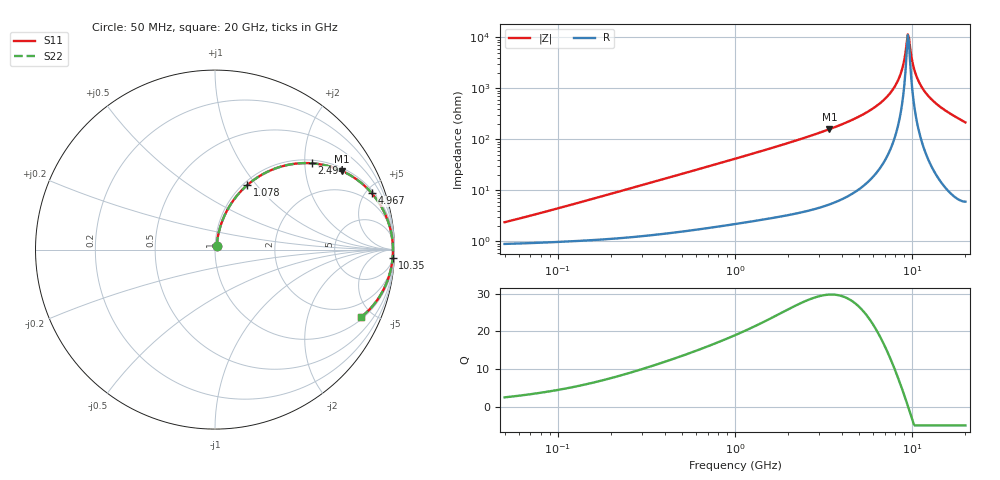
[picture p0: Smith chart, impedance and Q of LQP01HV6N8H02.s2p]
!Murata Part Number: LQP01HV6N8H02
!These Parameters are Measured in Series Mode Connection
!  o--[Z]--o
!Port1  Port2
!  o-------o
!Freq. Start=50[MHz] Stop=20[GHz], 401[Steps]
# Hz S RI R 50
!Freq.(Hz) S11(Real) S11(Imag) S21(Real) S21(Imag) S12(Real) S12(Imag) S22(Real) S22(Imag)
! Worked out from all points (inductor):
!   401 points, 50 MHz to 20 GHz, reference 50 ohm
!   read as one part in series: L = 6.94 nH near 62.6 MHz
!   highest Q = 29.8 at 3.415 GHz (marker M1), where L = 7.36 nH
!   self-resonance near 9.457 GHz
!   S11 on the Smith chart (normalised r, x): 50 MHz: 1.02, +0.04; 1.078 GHz: 1.05, +0.90; 2.494 GHz: 1.08, +2.16; 4.967 GHz: 1.21, +5.49; 10.35 GHz: 9, -43; 20 GHz: 1.12, -4.29
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5e7  0.00933 0.0216  0.9907 -0.0216  0.9907 -0.0216  0.00933 0.0216
1.364002e8  0.0135 0.0573  0.9865 -0.0573  0.9865 -0.0573  0.0135 0.0573
3.721004e8  0.0366 0.1489  0.9634 -0.1489  0.9634 -0.1489  0.0366 0.1489
1e9  0.1602 0.3414  0.8398 -0.3414  0.8398 -0.3414  0.1602 0.3414
1.077769e9  0.1796 0.3592  0.8204 -0.3592  0.8204 -0.3592  0.1796 0.3592
2.493527e9  0.5384 0.481  0.4616 -0.481  0.4616 -0.481  0.5384 0.481
2.728004e9  0.5876 0.4752  0.4124 -0.4752  0.4124 -0.4752  0.5876 0.4752
3.415248e9  0.7078 0.4383  0.2922 -0.4383  0.2922 -0.4383  0.7078 0.4383
4.966507e9  0.8738 0.3139  0.1262 -0.3139  0.1262 -0.3139  0.8738 0.3139
6.311513e9  0.9442 0.2061  0.0558 -0.2061  0.0558 -0.2061  0.9442 0.2061
7.442007e9  0.9743 0.1251  0.0257 -0.1251  0.0257 -0.1251  0.9743 0.1251
8.020766e9  0.9831 0.0872  0.0169 -0.0872  0.0169 -0.0872  0.9831 0.0872
8.516016e9  0.9879 0.0565  0.0121 -0.0565  0.0121 -0.0565  0.9879 0.0565
8.907419e9  0.9902 0.0333  0.00981 -0.0333  0.00981 -0.0333  0.9902 0.0333
9.316812e9  0.9914 0.00999  0.00863 -0.00999  0.00863 -0.00999  0.9914 0.00999
9.457416e9  0.9915 0.00221  0.00848 -0.00221  0.00848 -0.00221  0.9915 0.00221
9.745021e9  0.9914 -0.0134  0.00856 0.0134  0.00856 0.0134  0.9914 -0.0134
1.034674e10  0.9898 -0.0446  0.0102 0.0446  0.0102 0.0446  0.9898 -0.0446
1.131968e10  0.9835 -0.0914  0.0165 0.0914  0.0165 0.0914  0.9835 -0.0914
1.276073e10  0.9677 -0.1536  0.0323 0.1536  0.0323 0.1536  0.9677 -0.1536
1.550395e10  0.9225 -0.2526  0.0775 0.2526  0.0775 0.2526  0.9225 -0.2526
2e10  0.8146 -0.3748  0.1854 0.3748  0.1854 0.3748  0.8146 -0.3748
